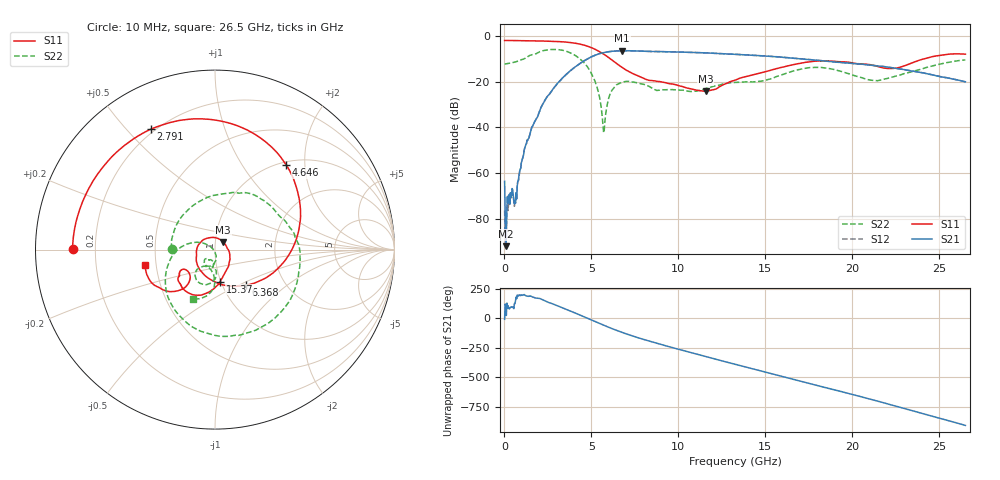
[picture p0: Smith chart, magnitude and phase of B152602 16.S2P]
!  2-Port S-parameters saved by WinCal
! VAR MeasName=S-Parameters (CALIBRATED_DATA) read from VNA (N5242A)
! VAR MeasDate=2016-1-5 16:27:33
! VAR NAME=B152602 16
! VAR FILENAME=B152602 16.S2P
! VAR DATE=2016-1-5 16:27:33
! VAR PHYS_PORTS=1,2
# Hz S DB R 50
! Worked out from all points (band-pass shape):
!   801 points, 10 MHz to 26.5 GHz, reference 50 ohm
!   highest |S21| = -6.48 dB at 6.765 GHz (marker M1); lowest = -91.8 dB at 76.22 MHz (marker M2)
!   |S21| within 3 dB of the highest: 4.918 GHz to 16.14 GHz (11.22 GHz wide, 107 % of centre)
!   lowest |S11| = -24.1 dB at 11.57 GHz (marker M3), VSWR 1.13, Z = 54.5 + j4.73 ohm
!   |S11| at or under -10 dB: 6.083 GHz to 24.14 GHz (18.05 GHz wide, 119 % of centre)
!   |S22| runs from -42.3 to -5.9 dB; largest |S21 - S12| = 0.0032
!   S11 on the Smith chart (normalised r, x): 10 MHz: 0.12, +0.00; 2.791 GHz: 0.18, +0.59; 4.646 GHz: 1.06, +1.61; 6.368 GHz: 1.28, -0.54; 15.37 GHz: 0.99, -0.37; 26.5 GHz: 0.43, -0.09
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1e7  -2.01 179.7  -63.50 -8.7  -76.17 10.3  -12.32 179.2
7.6225e7  -2.01 178.4  -91.81 104.4  -76.65 72.6  -12.24 173.3
6.391375e8  -2.07 166.8  -73.08 151.9  -72.23 148.8  -11.37 121.0
1.400725e9  -2.16 151.1  -44.75 -174.3  -44.81 -174.2  -8.77 59.9
2.162312e9  -2.26 134.0  -30.42 158.3  -30.45 158.3  -6.55 1.0
2.79145e9  -2.38 117.9  -23.19 121.3  -23.20 121.2  -5.93 -46.3
3.486812e9  -2.69 96.8  -17.30 79.7  -17.32 79.6  -6.58 -95.0
4.447075e9  -3.79 59.1  -11.53 21.0  -11.55 21.1  -10.79 -158.3
4.64575e9  -4.20 49.9  -10.59 8.6  -10.61 8.7  -12.30 -171.0
5.274888e9  -6.11 17.2  -8.27 -31.4  -8.27 -31.3  -21.27 153.5
5.70535e9  -7.99 -7.9  -7.32 -58.8  -7.31 -58.7  -42.32 -151.6
6.3676e9  -11.66 -49.3  -6.62 -98.1  -6.60 -98.0  -22.02 -94.6
6.76495e9  -13.76 -75.4  -6.48 -120.0  -6.47 -120.0  -20.25 -108.1
8.851038e9  -19.91 177.3  -6.86 144.5  -6.84 144.4  -23.77 -127.6
1.017554e10  -22.01 129.0  -7.10 90.5  -7.10 90.3  -23.71 -118.6
1.156626e10  -24.14 44.1  -7.43 35.0  -7.44 35.0  -22.99 -97.6
1.3255e10  -19.33 -42.9  -8.04 -30.0  -8.03 -30.0  -20.34 -98.5
1.53742e10  -14.88 -80.8  -9.00 -111.4  -8.98 -111.2  -18.60 -86.9
1.769208e10  -11.17 -113.2  -10.48 160.6  -10.45 160.6  -13.81 -107.5
1.967882e10  -11.40 -139.3  -11.84 86.3  -11.80 86.0  -16.28 -131.9
2.209604e10  -14.26 -141.8  -13.71 -9.0  -13.68 -9.3  -18.44 -98.9
2.65e10  -7.99 -167.7  -20.05 170.9  -20.06 170.6  -10.48 -113.7
